FUNCTION F_General : LREAL		// 使用直线的一般式方程
VAR_INPUT
    A, B, C: 		LREAL;  	// 直线方程系数 Ax + By + C = 0
    x0, y0: 		LREAL;  	// 点坐标
END_VAR
VAR
    Numerator:		LREAL;	// 分子
    Denominator:	LREAL;	// 分母
END_VAR

//计算分子：|Ax0 + By0 + C|
Numerator := ABS(A * x0 + B * y0 + C);

//计算分母：sqrt(A² + B²)
Denominator := SQRT(A * A + B * B);

//避免除零错误
IF Denominator = 0 THEN
    F_General := 0.0;
ELSE
    F_General := Numerator / denominator;
END_IF;

END_FUNCTION
